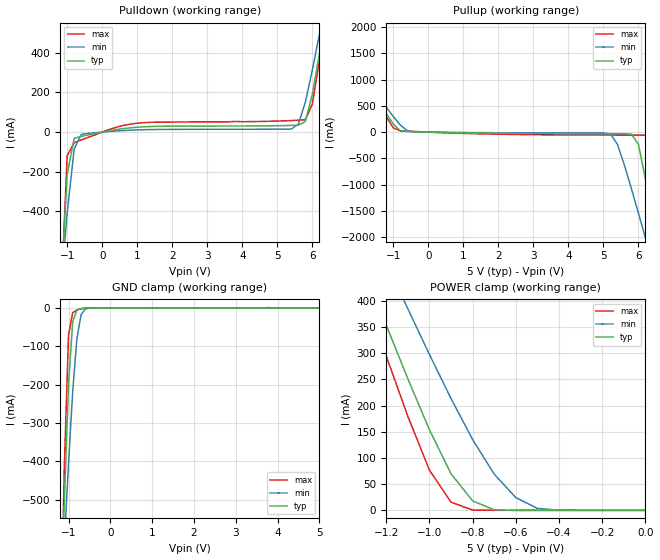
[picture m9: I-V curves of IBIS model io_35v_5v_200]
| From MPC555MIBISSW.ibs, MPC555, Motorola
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| io_35v_5v_200
[Model]   io_35v_5v_200
Model_type   I/O
Polarity   Non-Inverting
|   typ   min   max
C_comp   7.9550e-13   7.1400e-13   9.0400e-13
| CAP models
| typical : model= typ
| maximum : model= wcs
| minimum : model= bcs
[Voltage range]   5.0v   4.5v   5.5v
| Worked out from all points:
|   slope of the pulldown table from 0 to 0.75 V, typ, clamps not added: 36.8 ohm
|   slope of the pullup table from 0 to 0.75 V, typ, clamps not added: 64.3 ohm
|   GND clamp passes 1 mA (typ) near -0.66 V on its own axis
|   POWER clamp passes 1 mA (typ) near -0.69 V on its own axis
|  typical: model = typ,  temp = 25,  vdd = 5.0
|  maximum: model = bcs,  temp = -40, vdd = 5.5
|  minimum: model = wcs,  temp = 150, vdd = 4.5
[Pulldown]
|  Voltage   I(typ)   I(min)   I(max)
-5V       -16.37A    -10.07A    -25.06A
-1.2V     -865.7mA   -837.2mA   -953.5mA
-1V       -212.5mA   -408.3mA   -119.1mA
-800mV    -31.59mA   -86.23mA   -54.23mA
-600mV    -21.4mA    -11.76mA   -39.28mA
1V        24.56mA    10.89mA    44.97mA
5.4V      33.61mA    15.62mA    58.17mA
5.8V      53.76mA    151.5mA    62.77mA
6V        191.2mA    314.8mA    141.8mA
6.2V      392.7mA    491.9mA    362.9mA
6.4V      606.4mA    674.5mA    608.4mA
10V       4.688A     4.123A     5.338A
[GND_clamp]
-5V       -16.37A    -10.07A    -25.06A
-1.2V     -862.4mA   -836.3mA   -946.1mA
-1.1V     -505.3mA   -615.9mA   -414.3mA
-1V       -199.6mA   -406.4mA   -70.86mA
-900mV    -35.61mA   -218.7mA   -11.66mA
-800mV    -4.848mA   -79.69mA   -5.389mA
-700mV    -1.447mA   -17.89mA   -1.793mA
-600mV    -340.2uA   -2.494mA   -242uA
-500mV    -43.62uA   -353.5uA   -9.885uA
5V        119.7pA    22.38nA    107.4pA
[Pullup]
-5V       4.559A     4.065A     5.11A
-2.6V     1.885A     1.781A     2.05A
-800mV    25.61mA    136.4mA    23.39mA
5.2V      -32.01mA   -33.62mA   -56.34mA
5.8V      -37.34mA   -1.079A    -57.17mA
6V        -232.2mA   -1.544A    -57.42mA
6.2V      -895.2mA   -2.018A    -59.42mA
6.4V      -1.661A    -2.497A    -69.51mA
6.6V      -2.453A    -2.979A    -472.3mA
6.8V      -3.258A    -3.464A    -1.588A
7V        -4.069A    -3.95A     -2.808A
10V       -16.41A    -11.32A    -21.92A
[POWER_clamp]
-5V       4.559A     4.065A     5.11A
-1.3V     459.2mA    564.9mA    415.1mA
-1.2V     354.1mA    474.5mA    295.2mA
-1.1V     251.6mA    385.3mA    179.8mA
-1V       154.2mA    298mA      77.05mA
-900mV    70.04mA    213.8mA    15.71mA
-800mV    18.08mA    135.3mA    606.6uA
-700mV    1.079mA    69.19mA    104.9uA
-600mV    34.26uA    24.39mA    21.06uA
-500mV    2.117uA    3.8mA      1.676uA
-400mV    134.1nA    287.6uA    45.96nA
0V        119.7pA    21.86nA    118.6pA
| RAMP models
| typical dv/dt : model=typ, temp=25
| maximum dv/dt : model=bcs, temp=-40
| minimum dv/dt : model=wcs, temp=150
|		 typ   min   max
[Ramp]
dV/dt_r   1.35554/4.27378E-09   0.769416/3.51048E-09   3.04084/3.49565E-09
dV/dt_f   1.35554/4.52692E-09   0.769416/3.41165E-09   3.04084/3.91413E-09
